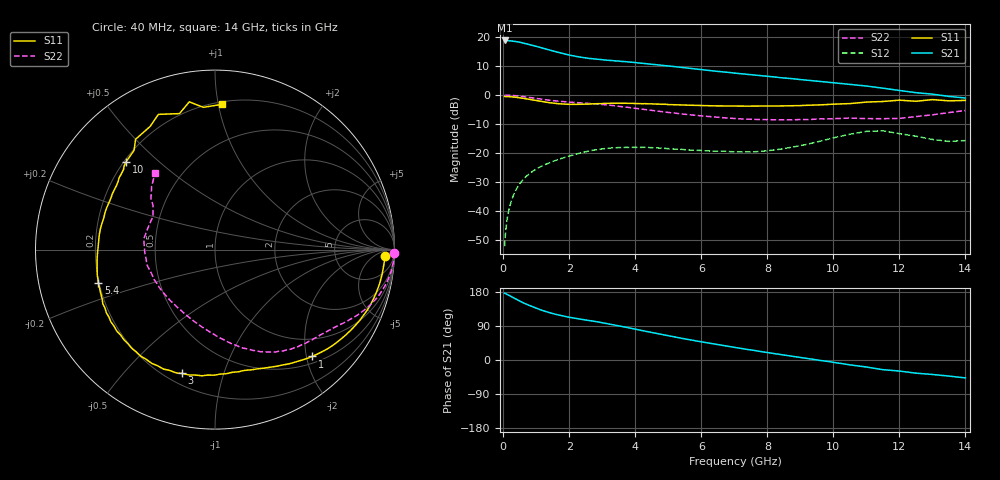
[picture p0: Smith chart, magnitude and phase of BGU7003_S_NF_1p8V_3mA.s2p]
!	Filename:	P:\Prog\Test\Noise\ATS_data\Testdata_Net\BGU7002	BGU7003	RN20082092\BGU7003_B1_high	freq_bias	loop_1.8V2.73mA_D.s2p
!	Date/Time:	Tue	16-Sep-08	9:20:17
!	BGU7003_B1_high	freq_bias	loop
!	bias	mode	1:00	Vout=	1.8002	"V,"	Iout=	2.723	"mA,"	Vin=	1.8402	"V,"	Iin=	0.2885	mA
!	Date/time	Wed	Aug	13	10:45:15	2008
!	Device	data	file	deembeded	for	feedlines	and	parallel
!	Original	file:	\BGU7002	BGU7003	RN20082092\BGU7003_B1_high	freq_bias	loop_1.8V2.73mA_R.s2p
!	Feed-files:	PR029V01_high	"frequency_140808_Feed1.s2p,"	PR029V01_high	frequency_140808_Feed2.s2p
!	Parallel-file:	PR029V01_high	frequency_140808_Par.s2p
#	MHz	S	MA	R	50
!	Freq-MHz	S11-mag	S11-arg	S21-mag	S21-arg	S12-mag	S12-arg	S22-mag	S22-arg
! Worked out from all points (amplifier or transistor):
!   144 points, 40 MHz to 14 GHz, reference 50 ohm
!   highest |S21| = 18.9 dB at 50 MHz (marker M1)
!   |S21| within 3 dB of that: start of sweep to 1.303 GHz
!   unconditionally stable (mu >= 1): nowhere
!   at 280 MHz: K = 0.09, MSG = 27.0 dB, |S12| = -35.4 dB
!   at 1.85 GHz: K = 0.40, MSG = 17.9 dB, |S12| = -21.6 dB
!   at 14 GHz: K = 0.76, MSG = 7.4 dB, |S12| = -15.7 dB
!   lowest NFmin = 0.42 dB at 400 MHz
!   S11 on the Smith chart (normalised r, x): 40 MHz: 25, -17; 1 GHz: 0.62, -2.11; 3 GHz: 0.26, -0.73; 5.4 GHz: 0.20, -0.13; 10 GHz: 0.21, +0.40; 14 GHz: 0.22, +1.02
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40  0.9473 -2.2  8.767 176.6  0.00246 89.3  0.9992 -1.1
50  0.9468 -2.7  8.782 175.9  0.00307 87.5  0.9991 -1.4
110  0.9438 -6.0  8.742 173.3  0.00677 86.6  0.9972 -3.2
220  0.9361 -11.9  8.635 168.4  0.01344 83.2  0.9908 -6.3
410  0.9125 -21.8  8.361 159.7  0.02453 77.3  0.971 -11.5
550  0.8881 -28.6  8.04 153.1  0.03218 73.3  0.9512 -15.1
750  0.8517 -37.7  7.568 145.4  0.04207 68.1  0.9174 -19.7
1000  0.8044 -47.8  6.949 136.6  0.05297 62.8  0.8752 -24.5
1200  0.7681 -54.9  6.473 130.3  0.0607 59.2  0.8426 -27.8
1600  0.716 -67.1  5.593 120.3  0.07497 53.5  0.7908 -33.5
2000  0.6924 -77.7  4.92 112.7  0.08868 48.1  0.7562 -38.8
2400  0.6943 -88.0  4.463 107.0  0.102 42.4  0.7303 -44.5
3000  0.7139 -105.0  4.07 98.3  0.1178 32.0  0.6867 -54.4
3700  0.7238 -124.6  3.784 86.7  0.1249 20.9  0.6233 -66.0
4700  0.6999 -149.8  3.318 68.9  0.1222 9.4  0.5264 -80.9
5400  0.6753 -164.2  3.008 57.3  0.1155 6.0  0.4726 -90.6
6200  0.6549 -178.3  2.678 45.0  0.1085 5.0  0.4276 -102.4
7200  0.6465 166.8  2.343 30.7  0.1045 7.7  0.3885 -118.9
9400  0.6711 141.1  1.764 1.6  0.1503 19.8  0.3821 -162.9
10000  0.6965 135.2  1.635 -6.0  0.1829 16.5  0.391 -176.6
12000  0.8168 112.7  1.202 -29.2  0.216 -24.4  0.3959 150.6
14000  0.8102 87.3  0.8907 -47.2  0.164 -27.2  0.5417 128.1
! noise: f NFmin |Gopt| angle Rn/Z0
400  0.42  0.51  13.27  0.2
1000  0.55  0.49  27.76  0.21
1500  0.67  0.48  39.83  0.2
1700  0.71  0.48  44.66  0.2
2200  0.82  0.47  56.73  0.19
3000  1  0.45  76.05  0.18
4400  1.32  0.45  109.8  0.13
5800  1.63  0.45  143.7  0.1
8000  2.12  0.49  -171.1  0.09
1.2e+04  3.02  0.66  -128.2  0.44
